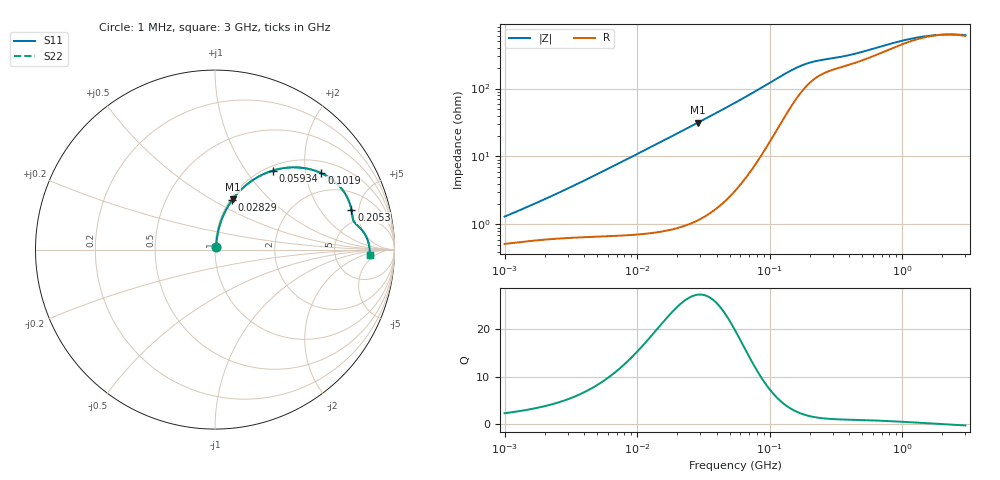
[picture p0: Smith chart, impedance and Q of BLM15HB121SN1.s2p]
! BLM15HB121SN1
# Hz S RI R 50
!Freq.(Hz) S11(Real) S11(Imag) S21(Real) S21(Imag) S12(Real) S12(Imag) S22(Real) S22(Imag)
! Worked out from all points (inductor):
!   401 points, 1 MHz to 3 GHz, reference 50 ohm
!   read as one part in series: L = 182 nH near 1.463 MHz
!   highest Q = 27.3 at 28.87 MHz (marker M1), where L = 174 nH
!   self-resonance near 2.137 GHz
!   S11 on the Smith chart (normalised r, x): 1 MHz: 1.01, +0.02; 28.29 MHz: 1.02, +0.62; 59.34 MHz: 1.07, +1.34; 101.9 MHz: 1.35, +2.45; 205.3 MHz: 3.52, +4.16; 3 GHz: 13, -3
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1000000  0.00528 0.0119  0.9947 -0.0119  0.9947 -0.0119  0.00528 0.0119
1859846  0.00631 0.021  0.9937 -0.021  0.9937 -0.021  0.00631 0.021
3823119  0.00816 0.0414  0.9918 -0.0414  0.9918 -0.0414  0.00816 0.0414
8017732  0.0142 0.0852  0.9858 -0.0852  0.9858 -0.0852  0.0142 0.0852
1.461624e7  0.0317 0.1524  0.9683 -0.1524  0.9683 -0.1524  0.0317 0.1524
2.829425e7  0.0958 0.2765  0.9042 -0.2765  0.9042 -0.2765  0.0958 0.2765
2.886629e7  0.0991 0.2811  0.9009 -0.2811  0.9009 -0.2811  0.0991 0.2811
4.05666e7  0.1771 0.3625  0.8229 -0.3625  0.8229 -0.3625  0.1771 0.3625
5.477226e7  0.2851 0.4269  0.7149 -0.4269  0.7149 -0.4269  0.2851 0.4269
5.933785e7  0.3205 0.4398  0.6795 -0.4398  0.6795 -0.4398  0.3205 0.4398
7.852918e7  0.4604 0.4577  0.5396 -0.4577  0.5396 -0.4577  0.4604 0.4577
1.018679e8  0.5925 0.4258  0.4075 -0.4258  0.4075 -0.4258  0.5925 0.4258
1.431579e8  0.7156 0.3259  0.2844 -0.3259  0.2844 -0.3259  0.7156 0.3259
2.052512e8  0.7604 0.2203  0.2396 -0.2203  0.2396 -0.2203  0.7604 0.2203
2.094008e8  0.7612 0.2158  0.2388 -0.2158  0.2388 -0.2158  0.7612 0.2158
2.942768e8  0.7699 0.1653  0.2301 -0.1653  0.2301 -0.1653  0.7699 0.1653
4.570858e8  0.7956 0.1327  0.2044 -0.1327  0.2044 -0.1327  0.7956 0.1327
8.005644e8  0.835 0.0861  0.165 -0.0861  0.165 -0.0861  0.835 0.0861
1.171007e9  0.8511 0.0517  0.1489 -0.0517  0.1489 -0.0517  0.8511 0.0517
1.613037e9  0.8585 0.0238  0.1415 -0.0238  0.1415 -0.0238  0.8585 0.0238
2.177892e9  0.8617 -0.00161  0.1383 0.00161  0.1383 0.00161  0.8617 -0.00161
3e9  0.8622 -0.0296  0.1378 0.0296  0.1378 0.0296  0.8622 -0.0296
